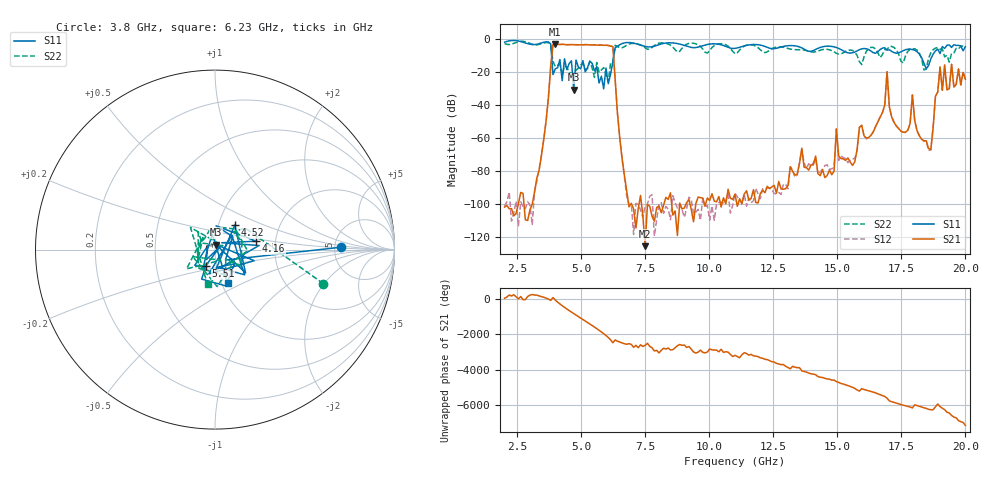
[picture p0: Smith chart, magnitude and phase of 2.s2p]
!Keysight Technologies,N5234A,MY52241180,A.10.60.03
!Date: Friday, January 20, 2023 09:32:59
!Correction: S11(Full 2 Port(1,2))
!S21(Full 2 Port(1,2))
!S12(Full 2 Port(1,2))
!S22(Full 2 Port(1,2))
!S2P File: Measurements: S11, S21, S12, S22:
# Hz S  dB  R 50
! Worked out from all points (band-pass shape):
!   201 points, 2 GHz to 20 GHz, reference 50 ohm
!   highest |S21| = -3.31 dB at 3.98 GHz (marker M1); lowest = -125.8 dB at 7.49 GHz (marker M2)
!   |S21| within 3 dB of the highest: 3.872 GHz to 6.237 GHz (2.365 GHz wide, 46.8 % of centre)
!   lowest |S11| = -30.8 dB at 4.7 GHz (marker M3), VSWR 1.06, Z = 50.4 + j2.86 ohm
!   |S11| at or under -10 dB: 3.833 GHz to 6.272 GHz (2.438 GHz wide, 48.3 % of centre); 18.23 GHz to 18.72 GHz (487.3 MHz wide, 2.64 % of centre)
!   |S22| runs from -26.2 to -1.5 dB; largest |S21 - S12| = 0.00032
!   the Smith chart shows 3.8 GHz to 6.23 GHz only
!   S11 on the Smith chart (normalised r, x): 3.8 GHz: 5.65, +0.28; 4.16 GHz: 1.59, +0.16; 4.52 GHz: 1.20, +0.34; 5.51 GHz: 0.89, -0.17; 6.23 GHz: 1.07, -0.42
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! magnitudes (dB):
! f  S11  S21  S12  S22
! 2 GHz  -2.1  -102.1  -101.6  -2.9
! 3.35 GHz  -2.9  -79.5  -78.9  -3.4
! 3.8 GHz  -3.1  -16.9  -16.9  -4.0
! 3.98 GHz  -18.3  -3.3  -3.3  -16.9
! 4.16 GHz  -12.6  -3.5  -3.5  -15.3
! 4.52 GHz  -15.1  -3.6  -3.6  -20.1
! 4.7 GHz  -30.8  -3.5  -3.5  -21.4
! 5.06 GHz  -13.3  -3.7  -3.7  -14.8
! 5.51 GHz  -19.4  -3.7  -3.7  -23.4
! 6.23 GHz  -14.0  -4.7  -4.7  -14.1
! 6.68 GHz  -2.5  -82.8  -83.9  -4.8
! 7.49 GHz  -4.6  -125.8  -101.2  -5.5
! 8.03 GHz  -3.5  -101.5  -100.1  -2.7
! 11 GHz  -5.8  -94.3  -93.6  -9.0
! 14.06 GHz  -7.2  -76.5  -75.2  -8.1
! 14.96 GHz  -5.3  -54.7  -54.8  -8.8
! 15.59 GHz  -8.5  -76.8  -73.0  -7.1
! 16.94 GHz  -6.8  -20.0  -20.0  -6.6
! 17.03 GHz  -6.7  -41.3  -41.3  -4.6
! 18.65 GHz  -12.2  -67.3  -67.3  -8.5
! 19.01 GHz  -9.0  -17.1  -17.1  -6.3
! 20 GHz  -4.8  -24.5  -24.5  -4.3
